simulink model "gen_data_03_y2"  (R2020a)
settings: Solver=ode45  StartTime=0.0  StopTime=3000  RelTol=1e-3  EnableMultiTasking=on
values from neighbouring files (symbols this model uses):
  Ts = 0.05    [init_model.m]

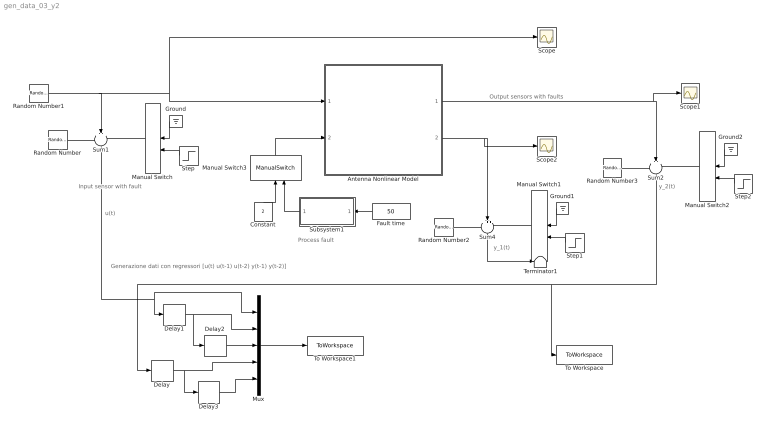
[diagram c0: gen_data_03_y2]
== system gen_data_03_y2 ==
  note: Generazione dati con regressori [u(t) u(t-1) u(t-2) y(t-1) y(t-2)]
  note: u(t)
  note: Output sensors with faults
  note: Process fault
  note: Input sensor with fault
  note: y_1(t)
  note: y_2(t)
  Antenna Nonlinear Model : Subsystem
  Constant : Constant  Value=2
  Delay{,1..3} (4 alike) : Delay  DelayLength=1  SampleTime=Ts
  Fault time : Constant  Value=50
  Ground : Ground
  Ground1 : Ground
  Ground2 : Ground
  Manual Switch{,1..3} (4 alike) : ManualSwitch
  Mux : Mux  Inputs=5
  Random Number : RandomNumber  Variance=0.0001  Seed=1  SampleTime=Ts
  Random Number1 : RandomNumber  Variance=0.1  SampleTime=10
  Random Number2 : RandomNumber  Variance=0.00001  Seed=2  SampleTime=Ts
  Random Number3 : RandomNumber  Variance=0.00001  Seed=3  SampleTime=Ts
  Scope : Scope
  Scope1 : Scope
  Scope2 : Scope
  Step : Step  Time=50  SampleTime=0
  Step1 : Step  Time=1500  SampleTime=0
  Step2 : Step  Time=50  SampleTime=0
  Subsystem1 : Subsystem
  Sum1 : Sum  Inputs=+++  SaturateOnIntegerOverflow=on
  Sum2 : Sum  Inputs=+++  SaturateOnIntegerOverflow=on
  Sum4 : Sum  Inputs=+++  SaturateOnIntegerOverflow=on
  Terminator1 : Terminator
  To Workspace : ToWorkspace  VariableName=Tsim  SampleTime=Ts
  To Workspace1 : ToWorkspace  VariableName=Psim  SampleTime=Ts
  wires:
  Random Number1/1 -> Scope/1, Antenna Nonlinear Model/1(force), Sum1/2
  Random Number/1 -> Sum1/1
  Manual Switch/1 -> Sum1/3
  Sum1/1 -> Delay1/1, Mux/1
  Ground/1 -> Manual Switch/1
  Step/1 -> Manual Switch/2
  Random Number2/1 -> Sum4/1
  Ground1/1 -> Manual Switch1/1
  Manual Switch1/1 -> Sum4/3
  Step1/1 -> Manual Switch1/2
  Antenna Nonlinear Model/2(velocity) -> Sum4/2, Scope2/1
  Random Number3/1 -> Sum2/1
  Ground2/1 -> Manual Switch2/1
  Manual Switch2/1 -> Sum2/3
  Step2/1 -> Manual Switch2/2
  Antenna Nonlinear Model/1(angle) -> Sum2/2, Scope1/1
  Sum2/1 -> To Workspace/1, Delay/1
  Fault time/1 -> Subsystem1/1(Fault time)
  Subsystem1/1(Fault) -> Manual Switch3/2
  Manual Switch3/1 -> Antenna Nonlinear Model/2(drag)
  Constant/1 -> Manual Switch3/1
  Mux/1 -> To Workspace1/1
  Delay1/1 -> Delay2/1, Mux/2
  Delay2/1 -> Mux/3
  Delay/1 -> Delay3/1, Mux/4
  Delay3/1 -> Mux/5
  Sum4/1 -> Terminator1/1

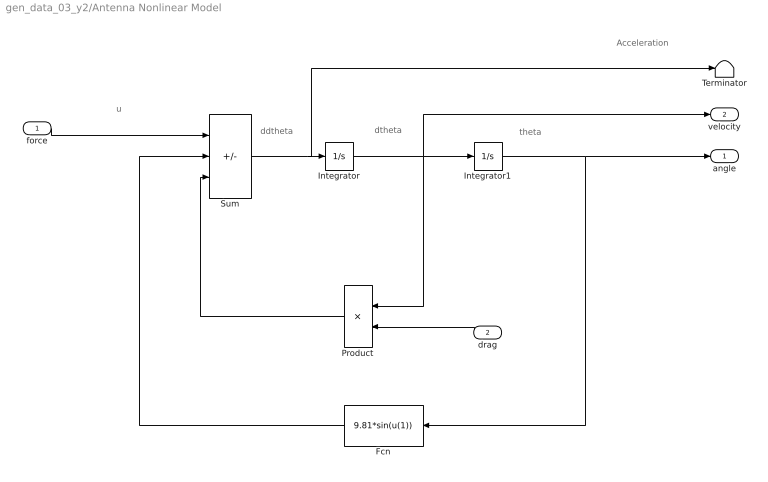
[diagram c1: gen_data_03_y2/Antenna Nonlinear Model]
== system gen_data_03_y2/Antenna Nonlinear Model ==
  note: Acceleration
  note: ddtheta
  note: dtheta
  note: theta
  note: u
  force : Inport
  drag : Inport  Port=2
  Fcn : Fcn  Expr=9.81*sin(u(1))
  Integrator : Integrator
  Integrator1 : Integrator  InitialCondition=(pi/180)*90
  Product : Product
  Sum : Sum  Inputs=+--  SaturateOnIntegerOverflow=on
  Terminator : Terminator
  angle : Outport
  velocity : Outport  Port=2
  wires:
  Sum/1 -> Terminator/1, Integrator/1
  Integrator/1 -> Product/1, Integrator1/1, velocity/1
  Integrator1/1 -> angle/1, Fcn/1
  Fcn/1 -> Sum/2
  Product/1 -> Sum/3
  force/1 -> Sum/1
  drag/1 -> Product/2

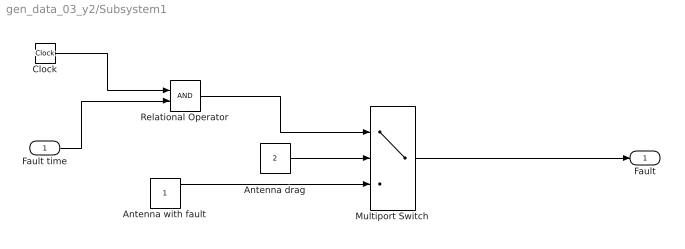
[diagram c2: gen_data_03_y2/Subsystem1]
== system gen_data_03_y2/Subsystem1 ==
  Fault time : Inport
  Antenna drag : Constant  Value=2
  Antenna with fault : Constant
  Clock : Clock
  Multiport Switch : MultiPortSwitch  DataPortOrder=Zero-based contiguous  Inputs=2  zeroidx=on
  Relational Operator : RelationalOperator  OutDataTypeStr=boolean  RndMeth=Simplest
  Fault : Outport
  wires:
  Clock/1 -> Relational Operator/1
  Fault time/1 -> Relational Operator/2
  Antenna drag/1 -> Multiport Switch/2
  Relational Operator/1 -> Multiport Switch/1
  Multiport Switch/1 -> Fault/1
  Antenna with fault/1 -> Multiport Switch/3
